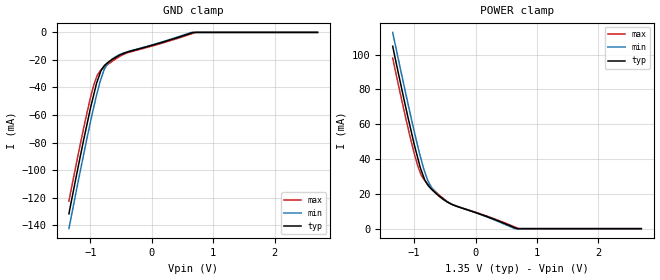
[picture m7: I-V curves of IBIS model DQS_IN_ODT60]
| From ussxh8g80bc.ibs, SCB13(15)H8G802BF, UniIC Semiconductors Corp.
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| MODEL DQS_IN_ODT60 (Data Strobe Input with 60ohm ODT, 800-2133Mbps)
[Model]   DQS_IN_ODT60
Model_type   Input
Vinl = 545.000mV
Vinh = 805.000mV
|   typ   min   max
|C_comp   1.069pF   1.013pF   1.108pF
C_comp_power_clamp   0.5345pF   0.5065pF   0.5540pF
C_comp_gnd_clamp   0.5345pF   0.5065pF   0.5540pF
| Note: C_comp changes when the ODT circuit is enabled.
[Model Spec]
| Input threshold voltage corners
Vinl   0.5450V   0.5115V   0.5825V
Vinh   0.8050V   0.7715V   0.8425V
| Dynamic Overshoot Parameters from DDR3L Specification
|D_overshoot_ampl_h   0.40   NA   NA
|D_overshoot_ampl_l   0.40   NA   NA
|D_overshoot_area_h   0.11n   NA   NA
|D_overshoot_area_l   0.11n   NA   NA
[Receiver Thresholds]
|Vth   =  0.675V
|Vth_min  =  0.6615V
|Vth_max  =  0.6885V
|Vinh_ac  =  0.130V
|Vinh_dc  =  0.090V
|Vinl_ac  = -0.130V
|Vinl_dc  = -0.090V
|Tslew_ac =  5.000ns |Not specified, so set to high value
|Threshold_sensitivity = 0.50
|Reference_supply Power_clamp_ref
|NOTE: If using the IBISCHK 4.2.1 or older parser, Differential receiver
|threshold parameters must be commented out because the parser generates
|errors for multiple differential models.
Vcross_low   = 0.545V
Vcross_high  = 0.805V
Vdiff_ac   = 260mV
Vdiff_dc   = 180mV
Tdiffslew_ac = 10.000ns |Not specified, so set to high value
[Voltage Range]   1.3500V   1.2830V   1.4250V
[POWER Clamp Reference]   1.3500V   1.2830V   1.4250V
| Junction Temperature (Ambient temp is 40C typ, 85C min, 0C max)
[Temperature Range]   45.0   90.0   0.0
[GND Clamp]
|   Voltage   I(typ)   I(min)   I(max)
-1.35V    -131.8mA   -142.6mA   -122.5mA
-1.11V    -77.97mA   -88.53mA   -69.42mA
-1V       -55.11mA   -65.16mA   -47.46mA
-945mV    -45.04mA   -54.11mA   -38.1mA
-885mV    -35.01mA   -42.95mA   -30.77mA
-825mV    -27.52mA   -33.34mA   -27.09mA
-780mV    -24.5mA    -27.42mA   -25.37mA
-715mV    -21.84mA   -22.34mA   -23.18mA
-650mV    -19.84mA   -19.53mA   -21.13mA
-410mV    -14.49mA   -14.22mA   -15.06mA
720mV     0A         0A         0A
2.7V      0A         0A         0A
[POWER Clamp]
|   Voltage   I(typ)   I(min)   I(max)
-1.35V    104.7mA    112.7mA    97.98mA
-1.11V    65.25mA    73.14mA    59.19mA
-940mV    40.31mA    47.08mA    35.85mA
-885mV    33.51mA    39.51mA    30.72mA
-830mV    28.17mA    32.8mA     27.62mA
-780mV    25.15mA    27.73mA    25.67mA
-715mV    22.52mA    23.42mA    23.36mA
-560mV    17.79mA    17.7mA     18.33mA
-335mV    13.18mA    13.33mA    13.27mA
640mV     509.7uA    0A         959.2uA
705mV     0A         0A         0A
2.7V      0A         0A         0A
